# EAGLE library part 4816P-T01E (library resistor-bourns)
BOURNS RESISTOR NETWORK
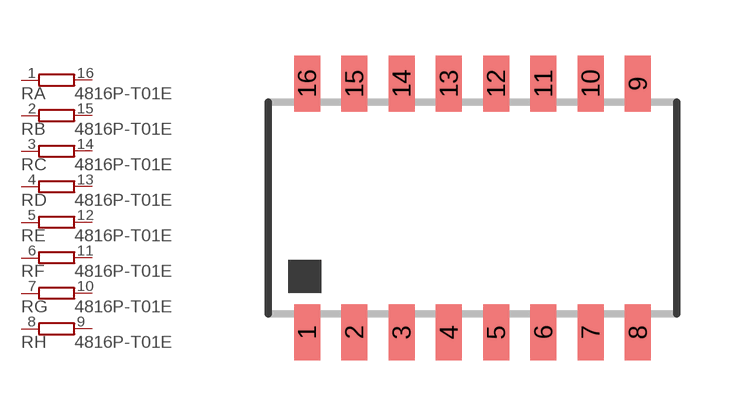
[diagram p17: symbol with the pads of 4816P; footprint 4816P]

Designator prefix R; gates A=R1NV B=R1NV C=R1NV D=R1NV E=R1NV F=R1NV G=R1NV H=R1NV

## 4816P-T01E (OC_FARNELL: unknown; OC_NEWARK: unknown)  [4816P]
1  A:1  pas
2  B:1  pas
3  C:1  pas
4  D:1  pas
5  E:1  pas
6  F:1  pas
7  G:1  pas
8  H:1  pas
9  H:2  pas
10  G:2  pas
11  F:2  pas
12  E:2  pas
13  D:2  pas
14  C:2  pas
15  B:2  pas
16  A:2  pas

## Footprint 4816P (pad centres in mm)
BOURNS RESISTOR NETWORK
smd 0.7 x 1.5: 1 -4.445,-3.346; 2 -3.175,-3.346; 3 -1.905,-3.346; 4 -0.635,-3.346; 5 0.635,-3.346; 6 1.905,-3.346; 7 3.175,-3.346; 8 4.445,-3.346; 9 4.445,3.346; 10 3.175,3.346; 11 1.905,3.346; 12 0.635,3.346; 13 -0.635,3.346; 14 -1.905,3.346; 15 -3.175,3.346; 16 -4.445,3.346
